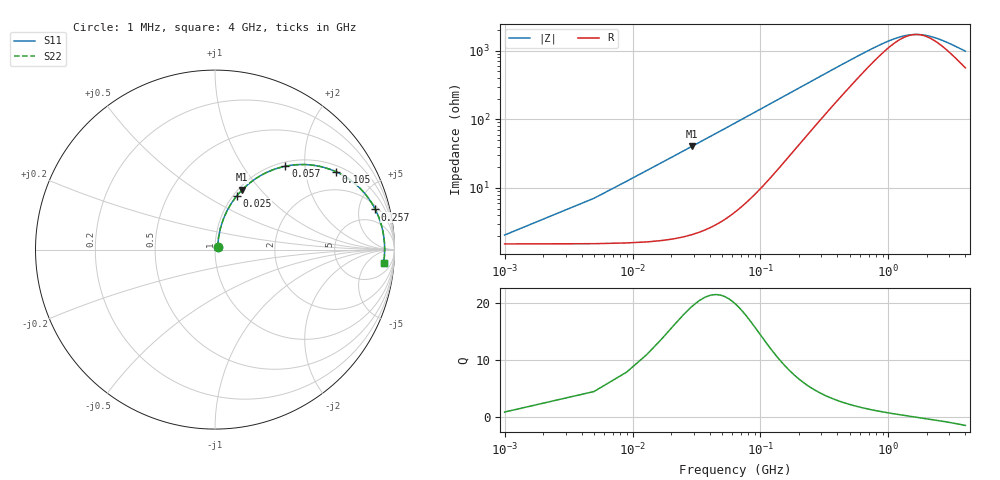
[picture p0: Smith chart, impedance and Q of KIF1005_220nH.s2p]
!version-2
!date-12.2020
!Series
# MHz S RI R 50
!Freq ReS11 ImS11 ReS21 ImS21 ReS12 ImS12 ReS22 ImS22
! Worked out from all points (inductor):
!   1001 points, 1 MHz to 4 GHz, reference 50 ohm
!   read as one part in series: L = 220 nH near 21 MHz
!   highest Q = 19 at 29 MHz (marker M1), where L = 220 nH
!   self-resonance near 1.654 GHz
!   S11 on the Smith chart (normalised r, x): 1 MHz: 1.03, +0.03; 25 MHz: 1.04, +0.69; 57 MHz: 1.08, +1.59; 105 MHz: 1.22, +2.95; 257 MHz: 2.47, +7.27; 4 GHz: 12, -16
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1  0.0152 0.0134  0.9848 -0.0134  0.9848 -0.0134  0.0152 0.0134
13  0.0459 0.1687  0.9541 -0.1687  0.9541 -0.1687  0.0459 0.1687
25  0.1203 0.2986  0.8797 -0.2986  0.8797 -0.2986  0.1203 0.2986
29  0.1517 0.3337  0.8483 -0.3337  0.8483 -0.3337  0.1517 0.3337
41  0.2547 0.4129  0.7453 -0.4129  0.7453 -0.4129  0.2547 0.4129
57  0.3919 0.4645  0.6081 -0.4645  0.6081 -0.4645  0.3919 0.4645
81  0.5596 0.4681  0.4404 -0.4681  0.4404 -0.4681  0.5596 0.4681
105  0.6749 0.4334  0.3251 -0.4334  0.3251 -0.4334  0.6749 0.4334
133  0.7607 0.3825  0.2393 -0.3825  0.2393 -0.3825  0.7607 0.3825
165  0.82 0.3291  0.18 -0.3291  0.18 -0.3291  0.82 0.3291
205  0.8628 0.2754  0.1372 -0.2754  0.1372 -0.2754  0.8628 0.2754
257  0.8931 0.224  0.1069 -0.224  0.1069 -0.224  0.8931 0.224
337  0.9159 0.1711  0.0841 -0.1711  0.0841 -0.1711  0.9159 0.1711
433  0.9285 0.1307  0.0715 -0.1307  0.0715 -0.1307  0.9285 0.1307
669  0.9397 0.0766  0.0603 -0.0766  0.0603 -0.0766  0.9397 0.0766
985  0.9438 0.0403  0.0562 -0.0403  0.0562 -0.0403  0.9438 0.0403
1337  0.9451 0.0159  0.0549 -0.0159  0.0549 -0.0159  0.9451 0.0159
1637  0.9453 0.000776  0.0547 -0.000776  0.0547 -0.000776  0.9453 0.000776
2001  0.945 -0.0142  0.055 0.0142  0.055 0.0142  0.945 -0.0142
2669  0.9437 -0.0369  0.0563 0.0369  0.0563 0.0369  0.9437 -0.0369
3337  0.9418 -0.0563  0.0582 0.0563  0.0582 0.0563  0.9418 -0.0563
4000  0.9393 -0.074  0.0607 0.074  0.0607 0.074  0.9393 -0.074
